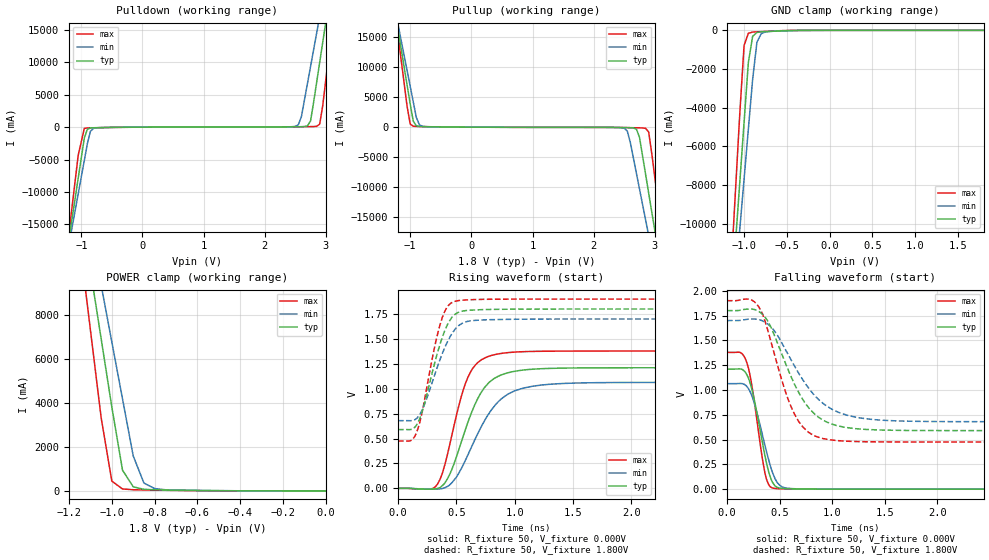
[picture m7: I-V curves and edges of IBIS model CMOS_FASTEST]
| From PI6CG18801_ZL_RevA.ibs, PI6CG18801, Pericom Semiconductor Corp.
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[Model]   CMOS_FASTEST
Model_type Output
Vref=1.800V
Vmeas=900mV
| variable   typ   min   max
C_comp   1.500pF   1.470pF   1.530pF
[Voltage Range]   1.8000V   1.7000V   1.9000V
[POWER Clamp Reference]   1.8000V   1.7000V   1.9000V
[GND Clamp Reference]   0.0000V   0.0000V   0.0000V
[Pullup Reference]   1.8000V   1.7000V   1.9000V
[Pulldown Reference]   0.0000V   0.0000V   0.0000V
[Temperature Range]   25   85   -40
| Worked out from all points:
|   slope of the pulldown table from 0 to 0.27 V, typ, clamps not added: 17.5 ohm
|   slope of the pullup table from 0 to 0.27 V, typ, clamps not added: 20 ohm
|   GND clamp passes 1 mA (typ) near -0.11 V on its own axis
|   POWER clamp passes 1 mA (typ) near -0.18 V on its own axis
|   falling waveform, R_fixture 50, V_fixture 0.000V: 20-80 % time 135ps typ, 154ps min, 115ps max; typ from 1.21 V to 0 V
|   rising waveform, R_fixture 50, V_fixture 0.000V: 20-80 % time 238ps typ, 295ps min, 185ps max; typ from 0 V to 1.21 V
|   falling waveform, R_fixture 50, V_fixture 1.800V: 20-80 % time 320ps typ, 382ps min, 256ps max; typ from 1.8 V to 0.59 V
|   rising waveform, R_fixture 50, V_fixture 1.800V: 20-80 % time 171ps typ, 194ps min, 148ps max; typ from 0.59 V to 1.8 V
[GND Clamp]
| Voltage   I(typ)   I(min)   I(max)
-1.8V     -54.41A    -49.04A    -63.81A
-1.15V    -14.08A    -15.46A    -12.25A
-1.1V     -10.97A    -12.87A    -8.279A
-1.05V    -7.872A    -10.29A    -4.312A
-1V       -4.77A     -7.709A    -788.1mA
-950mV    -1.668A    -5.127A    -151.5mA
-900mV    -312.3mA   -2.545A    -89.47mA
-850mV    -110.6mA   -620.5mA   -76.41mA
-800mV    -76.31mA   -175mA     -67.68mA
-750mV    -64.78mA   -80.98mA   -57.6mA
-300mV    -4.993mA   -4.79mA    -14.36uA
1.8V      310.7uA    609.2uA    13.92uA
[Power Clamp]
| Voltage   I(typ)   I(min)   I(max)
-1.8V     53.57A     48.2A      62.95A
-1.15V    13.13A     14.52A     11.28A
-1.1V     10.02A     11.93A     7.303A
-1.05V    6.913A     9.346A     3.331A
-1V       3.806A     6.758A     443mA
-950mV    940.8mA    4.171A     88.83mA
-900mV    186.8mA    1.586A     52.93mA
-850mV    72.78mA    357.1mA    44.07mA
-800mV    50.84mA    107.4mA    37.38mA
-750mV    41.62mA    52.42mA    30.27mA
-650mV    27.64mA    28.23mA    16.82mA
0V        310.7uA    425.9uA    14.69uA
[Pulldown]
| Voltage   I(typ)   I(min)   I(max)
-1.8V     -54.42A    -49.05A    -63.84A
-1.2V     -17.2A     -18.06A    -16.25A
-1.15V    -14.1A     -15.47A    -12.28A
-950mV    -1.689A    -5.144A    -191.1mA
-750mV    -87.68mA   -99.6mA    -100.8mA
2.55V     59.88mA    370.4mA    52.99mA
2.75V     956.7mA    9.357A     80.67mA
2.85V     6.928A     14.53A     125.7mA
2.9V      10.03A     17.12A     480mA
3V        16.25A     22.3A      7.34A
3.1V      22.47A     27.48A     15.29A
3.6V      53.58A     53.39A     55.04A
[Pullup]
| Voltage   I(typ)   I(min)   I(max)
-1.8V     53.63A     48.25A     63.06A
-1.25V    19.4A      19.74A     19.3A
-1.2V     16.29A     17.15A     15.33A
-1V       3.851A     6.797A     513.7mA
-950mV    984.1mA    4.208A     156.8mA
-800mV    86.58mA    137.9mA    94.43mA
2.5V      -78.71mA   -194.9mA   -67.08mA
2.7V      -336.9mA   -7.729A    -111.4mA
2.85V     -7.897A    -15.48A    -195.5mA
3V        -17.2A     -23.23A    -8.323A
3.1V      -23.41A    -28.39A    -16.26A
3.6V      -54.44A    -54.22A    -55.93A
[Falling Waveform]
R_fixture = 50
V_fixture = 0.000V
V_fixture_min = 0.000V
V_fixture_max = 0.000V
|   Time   V(typ)   V(min)   V(max)
0s        1.211V     1.064V     1.378V
132ps     1.211V     1.065V     1.375V
180ps     1.17V      1.045V     1.301V
252ps     939.1mV    894.2mV    941.5mV
336ps     475.4mV    551.7mV    312.2mV
372ps     282.2mV    394.8mV    114.5mV
420ps     98.9mV     208mV      18.12mV
480ps     16.97mV    64.26mV    5.39mV
960ps     548.7uV    968.1uV    261.1uV
20ns      8.716uV    9.649uV    8.201uV
[Rising Waveform]
R_fixture = 50
V_fixture = 0.000V
V_fixture_min = 0.000V
V_fixture_max = 0.000V
|   Time   V(typ)   V(min)   V(max)
0s        8.736uV    9.623uV    8.201uV
320ps     -5.945mV   -7.689mV   15.8mV
380ps     27.08mV    -1.781mV   150.8mV
440ps     131.7mV    31.34mV    421.9mV
560ps     528.5mV    238.6mV    991mV
640ps     789mV      441.5mV    1.204V
780ps     1.063V     752.7mV    1.326V
1.02ns    1.179V     986.4mV    1.369V
2ns       1.21V      1.063V     1.378V
20ns      1.211V     1.064V     1.378V
[Falling Waveform]
R_fixture = 50
V_fixture = 1.800V
V_fixture_min = 1.700V
V_fixture_max = 1.900V
|   Time   V(typ)   V(min)   V(max)
0s        1.8V       1.7V       1.9V
280ps     1.804V     1.713V     1.869V
340ps     1.76V      1.696V     1.762V
400ps     1.67V      1.654V     1.557V
560ps     1.259V     1.399V     970.3mV
680ps     978.8mV    1.172V     684.8mV
840ps     751mV      936.7mV    534.4mV
1.06ns    637.2mV    774mV      488.7mV
2.1ns     590.4mV    681.2mV    475.3mV
20ns      589.8mV    679.5mV    475mV
[Rising Waveform]
R_fixture = 50
V_fixture = 1.800V
V_fixture_min = 1.700V
V_fixture_max = 1.900V
|   Time   V(typ)   V(min)   V(max)
0s        589.8mV    679.5mV    475mV
110ps     590.4mV    678.9mV    479.9mV
160ps     637.3mV    702mV      562.6mV
220ps     822.2mV    821mV      842.2mV
330ps     1.326V     1.193V     1.503V
400ps     1.58V      1.409V     1.774V
480ps     1.739V     1.582V     1.874V
580ps     1.784V     1.67V      1.891V
1.4ns     1.8V       1.699V     1.9V
20ns      1.8V       1.7V       1.9V
[Ramp]
| variable   typ   min   max
dV/dt_r   0.72636V/238.03p   0.63822V/296.42p   0.82704V/185.14p
dV/dt_f   0.72589V/319.65p   0.61205V/381.31p   0.85482V/256.80p
R_load = 50
